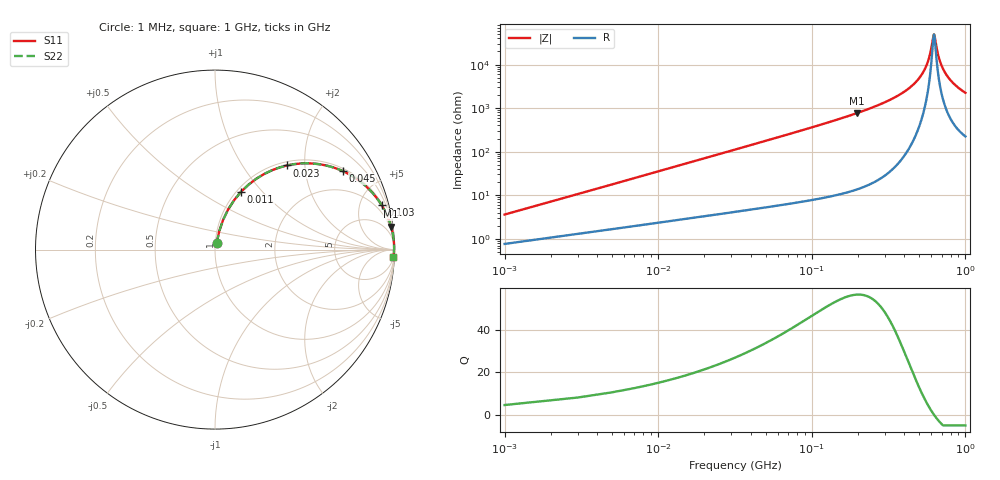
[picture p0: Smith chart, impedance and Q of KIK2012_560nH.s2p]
!version-2
!date-01.2022
!Series
# MHz S RI R 50
!Freq ReS11 ImS11 ReS21 ImS21 ReS12 ImS12 ReS22 ImS22
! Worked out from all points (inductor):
!   501 points, 1 MHz to 1 GHz, reference 50 ohm
!   read as one part in series: L = 560 nH near 5 MHz
!   highest Q = 56.7 at 197 MHz (marker M1), where L = 622 nH
!   self-resonance near 623 MHz
!   S11 on the Smith chart (normalised r, x): 1 MHz: 1.02, +0.07; 11 MHz: 1.05, +0.77; 23 MHz: 1.07, +1.62; 45 MHz: 1.10, +3.18; 103 MHz: 1.16, +7.45; 1 GHz: 5, -45
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1  0.00876 0.0346  0.9912 -0.0346  0.9912 -0.0346  0.00876 0.0346
7  0.0733 0.2239  0.9267 -0.2239  0.9267 -0.2239  0.0733 0.2239
11  0.1459 0.3228  0.8541 -0.3228  0.8541 -0.3228  0.1459 0.3228
17  0.2744 0.4216  0.7256 -0.4216  0.7256 -0.4216  0.2744 0.4216
23  0.4011 0.4688  0.5989 -0.4688  0.5989 -0.4688  0.4011 0.4688
45  0.7112 0.4379  0.2888 -0.4379  0.2888 -0.4379  0.7112 0.4379
69  0.8518 0.3428  0.1482 -0.3428  0.1482 -0.3428  0.8518 0.3428
103  0.9283 0.2477  0.0717 -0.2477  0.0717 -0.2477  0.9283 0.2477
169  0.9737 0.1513  0.0263 -0.1513  0.0263 -0.1513  0.9737 0.1513
197  0.9812 0.1272  0.0188 -0.1272  0.0188 -0.1272  0.9812 0.1272
335  0.9949 0.06  0.00506 -0.06  0.00506 -0.06  0.9949 0.06
501  0.998 0.0202  0.00199 -0.0202  0.00199 -0.0202  0.998 0.0202
541  0.9981 0.0131  0.00188 -0.0131  0.00188 -0.0131  0.9981 0.0131
571  0.9981 0.00818  0.00188 -0.00818  0.00188 -0.00818  0.9981 0.00818
591  0.9981 0.00506  0.00191 -0.00506  0.00191 -0.00506  0.9981 0.00506
623  0.998 0.000284  0.00202 -0.000284  0.00202 -0.000284  0.998 0.000284
631  0.9979 -0.00087  0.00206 0.00087  0.00206 0.00087  0.9979 -0.00087
667  0.9977 -0.00589  0.00226 0.00589  0.00226 0.00589  0.9977 -0.00589
695  0.9975 -0.00962  0.00246 0.00962  0.00246 0.00962  0.9975 -0.00962
731  0.9972 -0.0142  0.00276 0.0142  0.00276 0.0142  0.9972 -0.0142
835  0.9961 -0.0265  0.00389 0.0265  0.00389 0.0265  0.9961 -0.0265
1000  0.9937 -0.0437  0.00632 0.0437  0.00632 0.0437  0.9937 -0.0437
